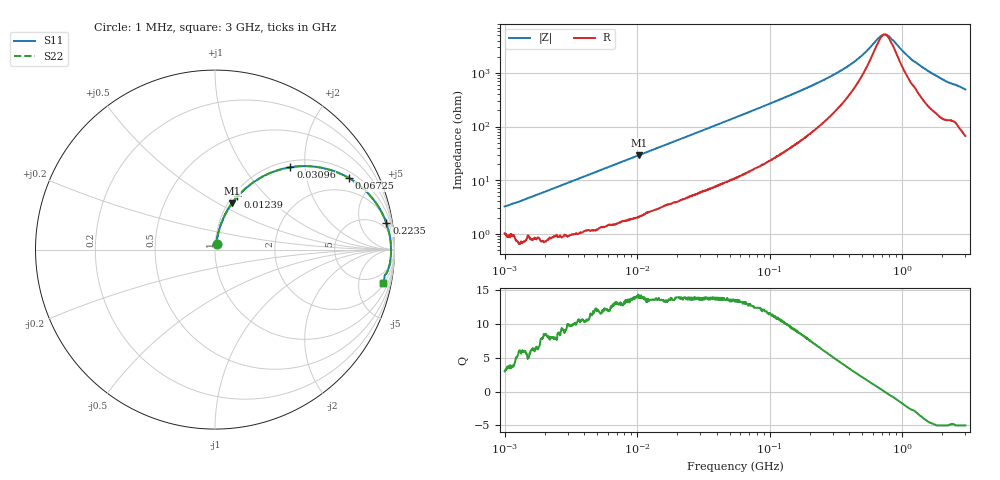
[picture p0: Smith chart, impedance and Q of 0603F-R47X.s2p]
!s-Parameter Generated by FASTRON Sdn. Bhd.
!FASTRON P/N : 0603F-R47X
!Keysight Technologies: E4991B_MY54100416_A.01.15
!Date: Thu Jun 20 13:32:14 2024
!Version  :Rev00  Thu Jun 20 13:32:14 2024
!Data & Calibration Information:
!Freq  S11  S21  S12  S22
!PortZ  Port1:50+j0  Port2:50+j0
!When reading reference impedance value at option line is always used.
! Remarks : This data is being provided solely for informational purposes.
# Hz S dB R 50
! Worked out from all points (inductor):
!   1601 points, 1 MHz to 3 GHz, reference 50 ohm
!   read as one part in series: L = 483 nH near 1.041 MHz
!   highest Q = 14 at 10.3 MHz (marker M1), where L = 450 nH
!   self-resonance near 737.6 MHz
!   S11 on the Smith chart (normalised r, x): 1 MHz: 1.02, +0.06; 12.39 MHz: 1.05, +0.69; 30.96 MHz: 1.12, +1.68; 67.25 MHz: 1.27, +3.57; 223.5 MHz: 3, +12; 3 GHz: 2.31, -9.65
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1000000  -29.90 69.9  -0.09 -1.7  -0.09 -1.7  -29.90 69.9
3804036  -19.20 78.3  -0.14 -6.3  -0.14 -6.3  -19.20 78.3
1.029702e7  -11.20 70.1  -0.52 -15.9  -0.52 -15.9  -11.20 70.1
1.239139e7  -9.86 67.1  -0.69 -18.7  -0.69 -18.7  -9.86 67.1
1.447069e7  -8.75 64.5  -0.87 -21.4  -0.87 -21.4  -8.75 64.5
2.064365e7  -6.38 57.3  -1.47 -28.6  -1.47 -28.6  -6.38 57.3
3.096105e7  -4.13 47.5  -2.62 -38.3  -2.62 -38.3  -4.13 47.5
5.504702e7  -1.94 32.9  -5.29 -52.9  -5.29 -52.9  -1.94 32.9
6.724529e7  -1.45 28.1  -6.51 -57.5  -6.51 -57.5  -1.45 28.1
1.131553e8  -0.68 17.8  -10.30 -67.0  -10.30 -67.0  -0.68 17.8
2.083556e8  -0.32 9.5  -15.60 -72.8  -15.60 -72.8  -0.32 9.5
2.234756e8  -0.30 8.8  -16.30 -73.0  -16.30 -73.0  -0.30 8.8
3.220132e8  -0.22 5.5  -20.20 -72.5  -20.20 -72.5  -0.22 5.5
4.32606e8  -0.19 3.3  -24.30 -68.0  -24.30 -68.0  -0.19 3.3
5.232078e8  -0.17 2.1  -27.70 -60.1  -27.70 -60.1  -0.17 2.1
6.993907e8  -0.17 0.3  -34.10 -16.2  -34.10 -16.2  -0.17 0.3
7.463997e8  -0.17 -0.1  -34.50 3.7  -34.50 3.7  -0.17 -0.1
7.925923e8  -0.17 -0.4  -33.80 21.7  -33.80 21.7  -0.17 -0.4
1.147801e9  -0.18 -2.8  -25.70 65.8  -25.70 65.8  -0.18 -2.8
1.423359e9  -0.19 -4.2  -22.30 71.1  -22.30 71.1  -0.19 -4.2
2.092429e9  -0.30 -7.6  -17.40 71.7  -17.40 71.7  -0.30 -7.6
3e9  -0.40 -11.2  -14.20 71.0  -14.20 71.0  -0.40 -11.2
